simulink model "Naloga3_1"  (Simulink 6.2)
settings: Solver=ode45  StartTime=0.0  StopTime=1  RelTol=1e-3
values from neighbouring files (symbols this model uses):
  f = 2250    [auto_param.m]    (also in auto_param_opt.m = 4500; basic_control_1.m = 0.2; cf.m = y(nt); cf_primer4_11.m = y(nt))
  k1 = 7500    [auto_param.m]    (also in auto_param_opt.m = 15000; Naloga31.m = 500; INTEG_RK4.M = krm(2)*DERIV(t,y,par); kovinska_palica_2_RK4.m = 10)
  k2 = 150000    [auto_param.m]    (also in auto_param_opt.m; Naloga31.m = 50000; INTEG_RK4.M = krm(2)*DERIV(t+0.5*krm(2),y+0.5*k1,par); kovinska_palica_2_RK4.m = 0.5)
  m1 = 500    [Naloga31.m]    (also in ex12_2st.m = 10; set_x4a.m = 1; za_podmodel_voz.m = 1)
  m2 = 10    [Naloga31.m]    (also in ex12_2st.m = 5; set_x4a.m = 3; za_podmodel_voz.m = 3)
  z = zero(pr_f_tf)    [basic_control_1.m]    (also in Naloga31.m = 0.1)

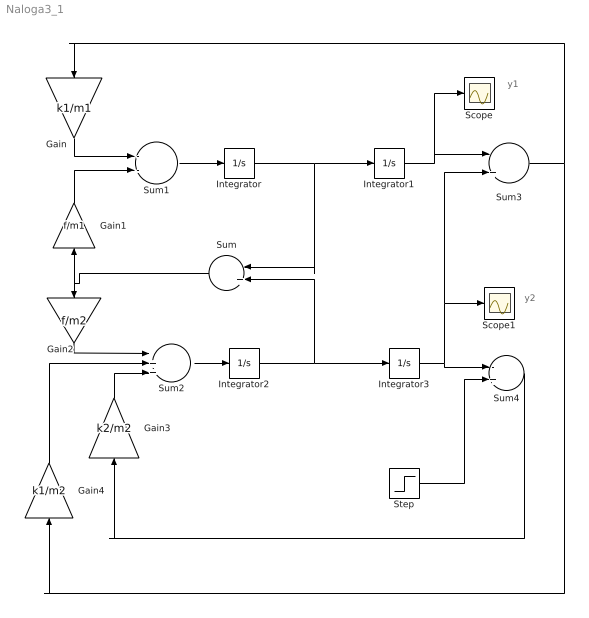
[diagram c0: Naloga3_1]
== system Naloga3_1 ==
  note: y1
  note: y2
  Gain : Gain  Orientation=down  Gain=k1/m1
  Gain1 : Gain  Orientation=up  Gain=f/m1
  Gain2 : Gain  Orientation=down  Gain=f/m2
  Gain3 : Gain  Orientation=up  Gain=k2/m2
  Gain4 : Gain  Orientation=up  Gain=k1/m2
  Integrator{,1..3} (4 alike) : Integrator
  Scope : Scope
  Scope1 : Scope
  Step : Step  Time=0  After=z  SampleTime=0
  Sum : Sum  Orientation=left  Inputs=|+-
  Sum1 : Sum  Inputs=--
  Sum2 : Sum  Inputs=|+++
  Sum3 : Sum  Inputs=|+-
  Sum4 : Sum  Inputs=-+
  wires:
  Sum1/1 -> Integrator/1
  Integrator1/1 -> Sum3/1, Scope/1
  Integrator2/1 -> Integrator3/1, Sum/2
  Integrator3/1 -> Sum4/1, Sum3/2, Scope1/1
  Sum2/1 -> Integrator2/1
  Sum3/1 -> Gain/1, Gain4/1
  Gain/1 -> Sum1/1
  Sum/1 -> Gain1/1, Gain2/1
  Gain1/1 -> Sum1/2
  Gain2/1 -> Sum2/1
  Sum4/1 -> Gain3/1
  Gain3/1 -> Sum2/3
  Gain4/1 -> Sum2/2
  Step/1 -> Sum4/2
  Integrator/1 -> Integrator1/1, Sum/1
